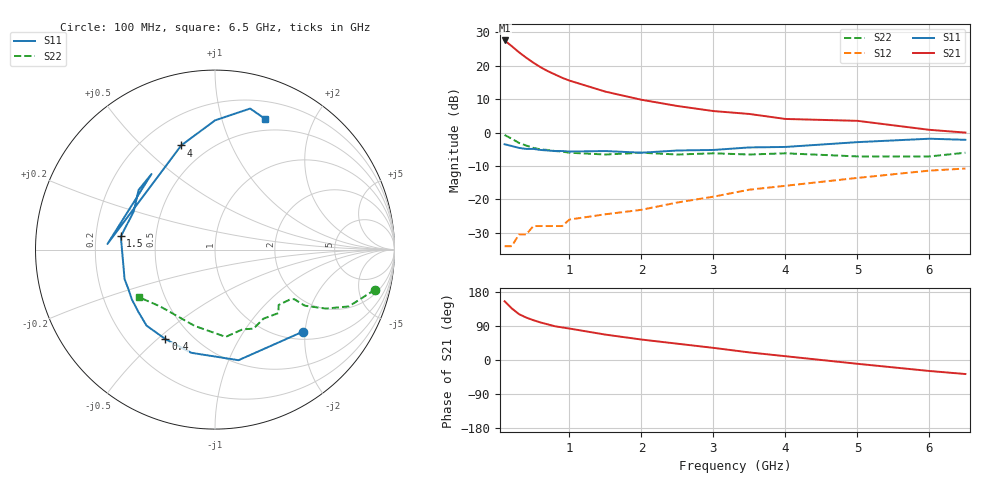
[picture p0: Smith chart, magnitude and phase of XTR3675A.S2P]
! HXTR-3675 Common Emitter
! Vce=10V  Ic=10mA
# ghz s ma r 50
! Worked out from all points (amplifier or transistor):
!   19 points, 100 MHz to 6.5 GHz, reference 50 ohm
!   highest |S21| = 27.6 dB at 100 MHz (marker M1)
!   |S21| within 3 dB of that: start of sweep to 270.3 MHz
!   unconditionally stable (mu >= 1): 1.462 GHz to 3.038 GHz
!   at 400 MHz: K = 0.45, MSG = 26.4 dB, |S12| = -30.5 dB
!   at 1 GHz: K = 0.83, MSG = 20.8 dB, |S12| = -26.0 dB
!   at 6.5 GHz: K = 0.51, MSG = 5.4 dB, |S12| = -10.8 dB
!   lowest NFmin = 1.20 dB at 1 GHz
!   S11 on the Smith chart (normalised r, x): 100 MHz: 1.18, -1.95; 400 MHz: 0.36, -0.53; 1.5 GHz: 0.31, +0.06; 4 GHz: 0.36, +0.66; 6.5 GHz: 0.37, +1.39
0.1  0.67 -43.0  23.9 155.0  0.02 66.0  0.92 -14.0
0.2  0.63 -78.0  19.6 136.0  0.02 70.0  0.81 -23.0
0.3  0.59 -103.0  15.9 121.0  0.03 53.0  0.7 -28.0
0.4  0.57 -119.0  13.2 112.0  0.03 52.0  0.64 -30.0
0.5  0.57 -132.0  11.1 105.0  0.04 46.0  0.59 -32.0
0.6  0.55 -141.0  9.5 99.0  0.04 49.0  0.56 -32.0
0.7  0.54 -149.0  8.3 94.0  0.04 50.0  0.55 -32.0
0.8  0.53 -156.0  7.4 89.0  0.04 49.0  0.53 -32.0
0.9  0.53 -162.0  6.6 86.0  0.04 51.0  0.52 -32.0
1  0.52 -168.0  6 83.0  0.05 50.0  0.5 -34.0
1.5  0.53 172.0  4.1 67.0  0.06 55.0  0.47 -41.0
2  0.5 155.0  3.1 54.0  0.07 58.0  0.5 -45.0
2.5  0.54 142.0  2.5 43.0  0.09 59.0  0.47 -55.0
3  0.55 130.0  2.1 32.0  0.11 58.0  0.49 -64.0
3.5  0.6 177.0  1.9 20.0  0.14 56.0  0.47 -71.0
4  0.61 108.0  1.6 10.0  0.16 52.0  0.49 -83.0
5  0.72 90.0  1.5 -10.0  0.21 43.0  0.44 -105.0
6  0.81 76.0  1.1 -29.0  0.27 32.0  0.44 -134.0
6.5  0.78 69.0  1 -37.0  0.29 26.0  0.5 -148.0
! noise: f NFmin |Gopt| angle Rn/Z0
1  1.2  0.2  135  0.13
2  1.8  0.4  -177  0.058
4  2.8  0.6  -117  0.43
